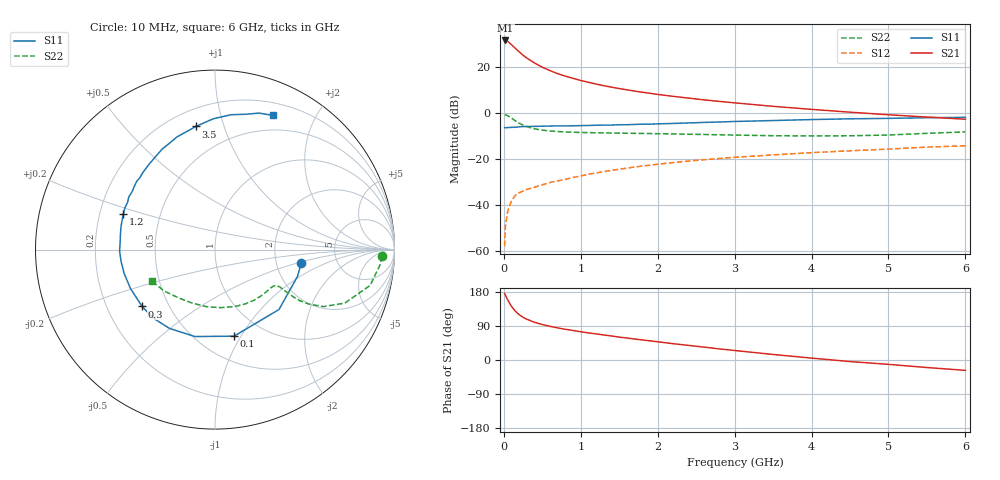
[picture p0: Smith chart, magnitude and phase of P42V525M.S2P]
! SIEMENS Small Signal Semiconductors
! BFP182
! Si NPN RF Bipolar Junction Transistor in SOT143
! VCE = 2.5 V  IC = 25 mA
! Common Emitter S-Parameters:  March  1996
# GHz  S  MA  R  50
!  f  S11  S21  S12  S22
! GHz  MAG  ANG  MAG  ANG  MAG  ANG  MAG  ANG
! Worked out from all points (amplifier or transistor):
!   36 points, 10 MHz to 6 GHz, reference 50 ohm
!   highest |S21| = 31.6 dB at 20 MHz (marker M1)
!   |S21| within 3 dB of that: start of sweep to 136.3 MHz
!   unconditionally stable (mu >= 1): start of sweep to 10.37 MHz; 517.4 MHz to 5.726 GHz
!   at 250 MHz: K = 0.64, MSG = 29.5 dB, |S12| = -33.8 dB
!   at 1.4 GHz: K = 1.31, MAG = 14.7 dB, |S12| = -24.8 dB
!   at 6 GHz: K = 0.98, MSG = 5.8 dB, |S12| = -14.1 dB
!   S11 on the Smith chart (normalised r, x): 10 MHz: 2.77, -0.55; 100 MHz: 0.73, -0.94; 300 MHz: 0.35, -0.30; 1.2 GHz: 0.30, +0.17; 3.5 GHz: 0.31, +0.81; 6 GHz: 0.33, +1.47
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0.01  0.486 -8.9  37.99 175.5  0.0013 83.5  0.9308 -2.3
0.02  0.4835 -18.0  38.04 171.4  0.0035 82.5  0.924 -5.2
0.05  0.4884 -43.1  36.16 158.6  0.0074 75.7  0.8869 -13.0
0.1  0.4939 -77.6  30.73 141.4  0.0126 62.6  0.7824 -22.4
0.15  0.4971 -103.0  25.62 128.6  0.0165 55.3  0.683 -27.7
0.2  0.5072 -120.0  21.49 119.5  0.0188 53.1  0.607 -30.1
0.25  0.5137 -132.0  18.21 112.6  0.0204 50.0  0.5509 -31.1
0.3  0.5151 -142.1  15.76 107.5  0.0222 49.9  0.5091 -31.1
0.4  0.5184 -155.3  12.3 99.4  0.0248 50.6  0.4588 -30.6
0.5  0.5235 -165.4  9.977 93.6  0.028 50.8  0.4295 -30.1
0.6  0.5277 -173.1  8.437 88.8  0.0313 52.8  0.4121 -30.0
0.7  0.5316 -179.2  7.226 84.7  0.034 54.2  0.401 -30.2
0.8  0.5299 175.8  6.385 81.0  0.0367 55.3  0.393 -30.7
1.1  0.5428 162.4  4.696 71.5  0.0474 56.3  0.3792 -33.6
1.2  0.5487 158.6  4.297 68.9  0.0505 56.2  0.3759 -34.9
1.7  0.5713 141.8  3.028 55.4  0.068 54.9  0.3656 -42.8
2.2  0.6002 128.0  2.327 43.1  0.0849 51.8  0.3562 -52.4
2.8  0.6449 113.1  1.809 29.3  0.1041 46.5  0.3397 -66.0
3.5  0.6944 98.8  1.413 14.6  0.1247 40.4  0.3251 -84.4
4.5  0.7568 83.2  1.054 -4.1  0.1531 31.8  0.3241 -113.3
5.5  0.7993 72.1  0.827 -19.9  0.184 23.1  0.3664 -141.2
6  0.8143 66.6  0.742 -27.3  0.1963 17.9  0.3935 -153.8
